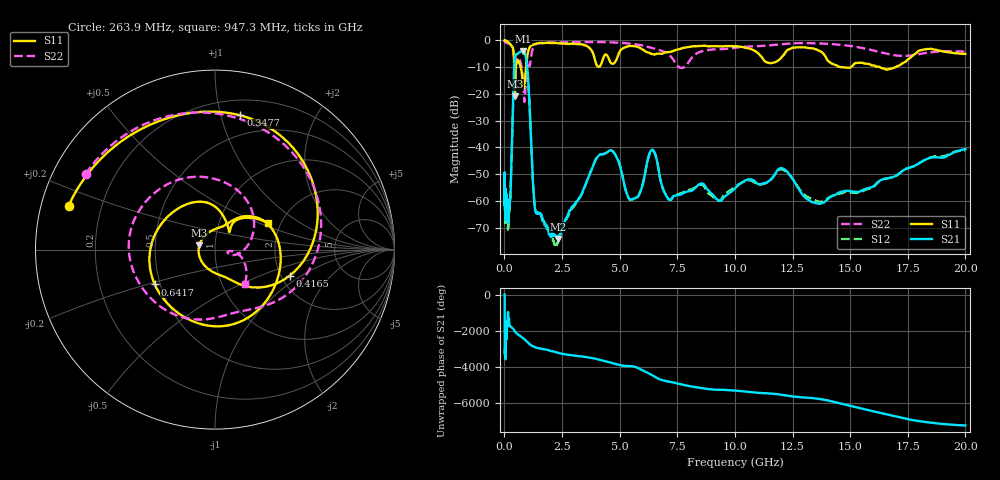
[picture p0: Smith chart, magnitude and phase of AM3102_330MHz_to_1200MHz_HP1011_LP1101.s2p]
! Date/Time: Tue, Sep 11, 2018 5:20 PM
! Network Analyzer: Agilent Technologies E8362B Rev: A.07.50.63
! Sweep from 0.010 to 20.000 GHz, 1601 Points, Sweep Type: LOG
! Power Supply: 4.949 V, 0.001 A
# Hz S DB R 50
!freq MagS11 AngS11 MagS21 AngS21 MagS12 AngS12 MagS22 AngS22
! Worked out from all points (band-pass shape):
!   1601 points, 10 MHz to 20 GHz, reference 50 ohm
!   highest |S21| = -3.89 dB at 798.4 MHz (marker M1); lowest = -74.2 dB at 2.336 GHz (marker M2)
!   |S21| within 3 dB of the highest: 451.1 MHz to 945.1 MHz (493.9 MHz wide, 70.8 % of centre)
!   lowest |S11| = -20.8 dB at 455.8 MHz (marker M3), VSWR 1.20, Z = 41.9 + j2.1 ohm
!   |S11| at or under -10 dB: 704.4 MHz to 942.6 MHz (238.2 MHz wide, 28.9 % of centre); 14.64 GHz to 15.03 GHz (386.8 MHz wide, 2.61 % of centre); 16.29 GHz to 16.96 GHz (663.7 MHz wide, 3.99 % of centre)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
!   |S22| runs from -23.0 to -0.2 dB; largest |S21 - S12| = 0.0095
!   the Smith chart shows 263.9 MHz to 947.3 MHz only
!   S11 on the Smith chart (normalised r, x): 263.9 MHz: 0.08, +0.14; 347.7 MHz: 0.32, +1.15; 416.5 MHz: 2.23, -0.80; 641.7 MHz: 0.47, -0.21; 947.3 MHz: 1.73, +0.58
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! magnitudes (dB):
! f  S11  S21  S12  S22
! 10 MHz  0.0  -49.8  -51.3  -0.2
! 35.55 MHz  0.0  -62.4  -68.7  -0.5
! 47.28 MHz  0.0  -57.5  -54.9  -0.6
! 126.4 MHz  -0.4  -65.9  -65.9  -1.0
! 263.9 MHz  -1.4  -57.2  -57.6  -1.6
! 347.7 MHz  -2.4  -32.7  -32.8  -2.6
! 416.5 MHz  -7.1  -12.2  -12.2  -5.7
! 447.2 MHz  -20.1  -7.2  -7.3  -8.3
! 455.8 MHz  -20.8  -6.6  -6.6  -8.6
! 641.7 MHz  -8.2  -4.5  -4.6  -6.8
! 798.4 MHz  -16.0  -3.9  -4.0  -14.1
! 947.3 MHz  -9.6  -7.0  -7.1  -11.9
! 1.309 GHz  -1.4  -61.5  -61.3  -1.8
! 1.59 GHz  -1.0  -65.2  -65.3  -0.9
! 2.336 GHz  -1.0  -74.2  -74.6  -0.7
! 4.171 GHz  -9.3  -42.7  -42.6  -0.6
! 5.652 GHz  -2.1  -59.1  -59.1  -1.4
! 6.396 GHz  -5.0  -40.9  -41.3  -2.8
! 7.202 GHz  -4.3  -59.6  -59.6  -5.8
! 12.03 GHz  -6.2  -47.7  -48.2  -1.4
! 13.55 GHz  -3.4  -60.9  -60.0  -1.1
! 20 GHz  -5.0  -40.6  -41.1  -4.2
